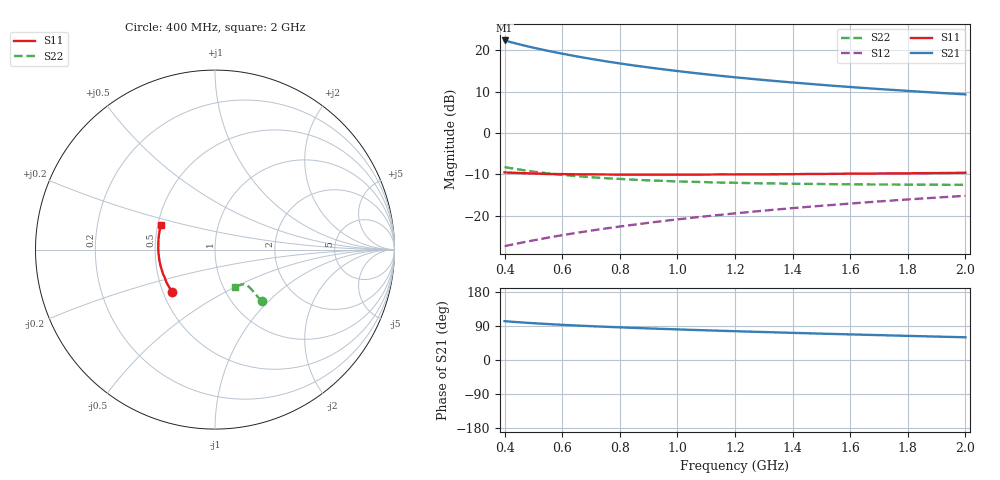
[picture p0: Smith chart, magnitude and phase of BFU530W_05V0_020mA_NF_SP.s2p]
! Filename:  P:\Prog\Test\Noise\ATS_data\Testdata_Net\06 Compressed Noise after Statistics\BFU530W_APM2013_09_A05_05p0V_020mA_NF_CM01_D.sf
! Date/Time: Tue 26/Mar/2013 18:06:04
! BFU530W_APM2013_09_A05_05p0V_1to25mA_NF_CM01_Bias8_R.sf
! Noise Parameter Data File
! BFU530W_APM2013_09_A05_05p0V_1to25mA_NF_CM01
! Date/time: Thu Mar 21 20:31:54 2013
! VAR V_out= 5.000000
! VAR I_out= 20.005000
! VAR V_in= 0.833100
! VAR I_in= 0.213750
! Device data file deembeded for feedlines and parallel
! Original file: \06 Compressed Noise after Statistics\BFU530W_APM2013_09_A05_05p0V_020mA_NF_CM01_R.sf
! Feed-files: PR019V01_070313_Feed1.s2p, PR019V01_070313_Feed2.s2p
! Parallel-file: PR019V01_070313_Par.s2p
# MHz S MA R 50
!  Freq-MHz  S11-mag  S11-arg  S21-mag  S21-arg  S12-mag  S12-arg  S22-mag  S22-arg
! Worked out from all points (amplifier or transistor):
!   37 points, 400 MHz to 2 GHz, reference 50 ohm
!   highest |S21| = 22.4 dB at 400 MHz (marker M1)
!   |S21| within 3 dB of that: start of sweep to 586 MHz
!   unconditionally stable (mu >= 1): 1.014 GHz to end of sweep
!   at 500 MHz: K = 0.89, MSG = 23.3 dB, |S12| = -25.9 dB
!   at 1.1 GHz: K = 1.01, MAG = 16.7 dB, |S12| = -20.1 dB
!   at 2 GHz: K = 1.01, MAG = 11.7 dB, |S12| = -15.2 dB
!   lowest NFmin = 0.99 dB at 433 MHz
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400  0.3351 -135.5  13.16 102.5  0.04304 65.8  0.389 -47.6
420  0.3325 -138.1  12.61 101.2  0.0445 66.1  0.3779 -47.8
440  0.3306 -140.4  12.09 100.1  0.04602 66.4  0.3677 -47.8
460  0.3287 -142.4  11.61 99.1  0.04756 66.7  0.3592 -47.8
500  0.3255 -146.6  10.76 97.1  0.05054 67.3  0.3426 -47.8
550  0.3202 -150.8  9.872 94.9  0.05451 68.0  0.3267 -47.6
600  0.32 -154.7  9.113 92.8  0.05844 68.5  0.3128 -47.6
650  0.3178 -158.2  8.454 91.0  0.06233 68.9  0.3024 -47.5
700  0.3167 -161.4  7.883 89.3  0.06632 69.3  0.2933 -47.6
750  0.3162 -164.2  7.385 87.7  0.0703 69.6  0.2852 -47.5
800  0.3153 -167.1  6.947 86.2  0.07436 69.8  0.2797 -47.8
850  0.3156 -169.6  6.559 84.7  0.07837 70.0  0.2732 -47.9
900  0.315 -171.8  6.213 83.4  0.08244 70.3  0.2684 -48.0
950  0.3149 -173.9  5.903 82.0  0.08658 70.4  0.2649 -48.4
1050  0.3155 -177.9  5.366 79.5  0.0948 70.5  0.2581 -49.0
1150  0.3167 178.3  4.92 77.1  0.103 70.4  0.2525 -49.9
1200  0.3164 176.7  4.728 76.0  0.1072 70.3  0.2512 -50.5
1350  0.3183 172.1  4.231 72.7  0.1198 70.0  0.2462 -52.2
1500  0.3209 167.6  3.83 69.5  0.1324 69.5  0.2427 -54.4
1650  0.3236 163.5  3.503 66.6  0.1451 68.9  0.24 -56.5
1750  0.3258 161.2  3.321 64.7  0.1536 68.4  0.2393 -58.1
2000  0.3321 155.1  2.936 59.9  0.1747 67.0  0.2377 -62.6
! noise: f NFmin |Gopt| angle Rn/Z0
400  1.005  0.2774  -172.5  0.0703
460  1.019  0.2777  -171.6  0.0702
600  1.008  0.2743  -169.9  0.0746
800  1.046  0.2886  -165.8  0.0748
1000  1.083  0.2966  -162.1  0.0738
1200  1.113  0.3061  -159.3  0.0765
1400  1.161  0.3138  -155.3  0.0812
1600  1.161  0.3203  -151.8  0.0846
1800  1.201  0.3502  -148.3  0.0823
2000  1.235  0.339  -145.5  0.094
